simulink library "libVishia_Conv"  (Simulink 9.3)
settings: Solver=ode45  StartTime=0.0  StopTime=10.0  RelTol=1e-3  EnableMultiTasking=on
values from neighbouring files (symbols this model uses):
  Tstep = 0.000050    (= 5e-05)    [TestOrthOsc_init.m]    (also in Test_PIDctrl_init.m = 0.0001)
undefined symbols (not defined in the file or in its folder): b0bit, b1bit, b2bit, b3bit, b4bit, b5bit, b6bit, b7bit, bit, Bitnr, hi, lo, maxFader, val, x0, xnom, y0, ynom
libraries: simulink x2

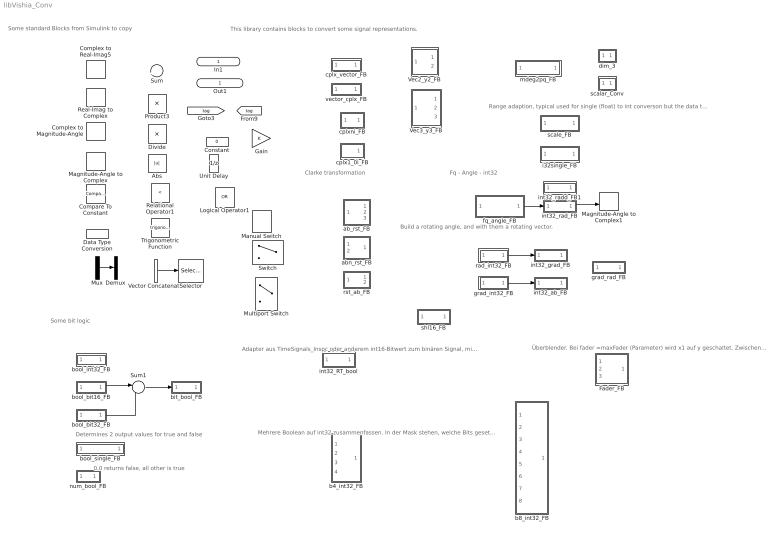
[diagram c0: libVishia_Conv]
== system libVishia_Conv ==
  note: Range adaption, typical used for single (float) to int converson but the data types on input and output depends on connected ones (forward and back propageted). Insert it is a data type conversion element.
  note: Some standard Blocks from Simulink to copy
  note: Mehrere Boolean auf int32 zusammenfassen. In der Mask stehen, welche Bits gesetzt werden. Default ist 0..3 bzw. 0..7, lässt sich ändern.
  note: Überblender. Bei fader =maxFader (Parameter) wird x1 auf y geschaltet. Zwischen diesen Werten überblenden.
  note: Adapter aus TimeSignals_Inspc oder anderem int16-Bitwert zum binären Signal, mit Angabe Bit-Nummer als Parameter. Einschließlich Rate-Transition, Ausgang kann in TstepHw direkt verwendet werden.
  note: This library contains blocks to convert some signal representations.
  note: Determines 2 output values for true and false
  note: 0.0 returns false, all other is true
  note: Clarke transformation
  note: Build a rotating angle, and with them a rotating vector.
  note: Fq - Angle - int32
  note: Some bit logic
  In1 : Inport  OutDataTypeStr=single  PortDimensions=1
  Abs : Abs
  Compare To Constant : simulink/Logic and Bit Operations/Compare To Constant  relop=<=  const=3.0  OutDataTypeStr=boolean
  Complex to Magnitude-Angle : ComplexToMagnitudeAngle
  Complex to Real-Imag5 : ComplexToRealImag
  Constant : Constant  Value=0  OutDataTypeStr=single
  Data Type Conversion : DataTypeConversion  OutDataTypeStr=int32
  Demux : Demux  Outputs=2
  Divide : Product  Inputs=*/
  Fader_FB : Subsystem
  Gain : Gain
  Logical Operator1 : Logic  Operator=OR  IconShape=distinctive  AllPortsSameDT=off  OutDataTypeStr=boolean
  Magnitude-Angle to Complex : MagnitudeAngleToComplex
  Magnitude-Angle to Complex1 : MagnitudeAngleToComplex
  Manual Switch : ManualSwitch
  Multiport Switch : MultiPortSwitch
  Mux : Mux  Inputs=2
  Product3 : Product
  Real-Imag to Complex : RealImagToComplex
  Relational Operator1 : RelationalOperator  Operator=<  OutDataTypeStr=boolean
  Selector : Selector  InputPortWidth=3  IndexOptions=Index vector (dialog)  Indices=[1 3]  OutputSizes=1
  Sum : Sum  Inputs=|++
  Sum1 : Sum  Inputs=|++
  Switch : Switch  Criteria=u2 > Threshold
  Trigonometric Function : Trigonometry
  Unit Delay : UnitDelay  SampleTime=-1  HasFrameUpgradeWarning=on
  Vec2_y2_FB : Subsystem
  Vec3_y3_FB : Subsystem
  Vector Concatenate : Concatenate
  ab_rst_FB : Subsystem
  abn_rst_FB : Subsystem
  b4_int32_FB : Subsystem
  b8_int32_FB : Subsystem
  bit_bool_FB : Subsystem
  bool_bit16_FB : Subsystem
  bool_bit32_FB : Subsystem
  bool_int32_FB : Subsystem
  bool_single_FB : Subsystem
  cplx1_0i_FB : Subsystem
  cplx_vector_FB : Subsystem
  cplxni_FB : Subsystem
  dim_3 : Subsystem
  fq_angle_FB : Subsystem
  grad_int32_FB : Subsystem  TreatAsAtomicUnit=on
  grad_rad_FB : Subsystem
  i32single_FB : Subsystem
  int32_RT_bool : Subsystem
  int32_ab_FB : Subsystem
  int32_grad_FB : Subsystem
  int32_rad_FB : Subsystem
  int32_radd_FB1 : Subsystem
  mdeg2pq_FB : Subsystem
  num_bool_FB : Subsystem
  rad_int32_FB : Subsystem  TreatAsAtomicUnit=on
  rst_ab_FB : Subsystem
  scalar_Conv : Subsystem
  scale_FB : Subsystem
  shl16_FB : Subsystem  TreatAsAtomicUnit=on
  vector_cplx_FB : Subsystem
  Out1 : Outport  OutDataTypeStr=single  PortDimensions=1
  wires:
  int32_rad_FB/1(Out1) -> Magnitude-Angle to Complex1/2
  fq_angle_FB/1(Gint32) -> int32_rad_FB/1(In1)
  rad_int32_FB/1(mwi) -> int32_grad_FB/1(In1)
  grad_int32_FB/1(mwi) -> int32_ab_FB/1(In1)
  Mux/1 -> Demux/1
  Vector Concatenate/1 -> Selector/1
  bool_bit16_FB/1(y) -> Sum1/1
  Sum1/1 -> bit_bool_FB/1(b)
  bool_bit32_FB/1(y) -> Sum1/2

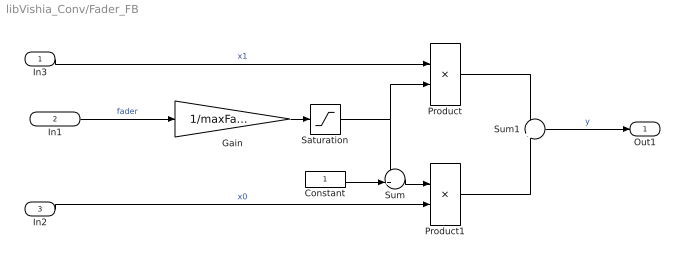
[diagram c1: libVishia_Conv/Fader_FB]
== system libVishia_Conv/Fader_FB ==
  In3 : Inport  OutDataTypeStr=single
  In1 : Inport  Port=2  OutDataTypeStr=single
  In2 : Inport  Port=3  OutDataTypeStr=single
  Constant : Constant  OutDataTypeStr=single
  Gain : Gain  Gain=1/maxFader
  Product : Product
  Product1 : Product
  Saturation : Saturate  UpperLimit=1  LowerLimit=0  ZeroCross=off
  Sum : Sum  Inputs=-+|
  Sum1 : Sum  Inputs=+|+
  Out1 : Outport  OutDataTypeStr=single
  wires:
  In1/1 -> Gain/1  "fader"
  Gain/1 -> Saturation/1
  Saturation/1 -> Product/2, Sum/1
  Constant/1 -> Sum/2
  Sum/1 -> Product1/1
  In2/1 -> Product1/2  "x0"
  In3/1 -> Product/1  "x1"
  Product/1 -> Sum1/1
  Product1/1 -> Sum1/2
  Sum1/1 -> Out1/1  "y"

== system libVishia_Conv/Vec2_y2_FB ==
  In1 : Inport  PortDimensions=2
  Selector : Selector  IndexMode=Zero-based  InputPortWidth=2  IndexOptions=Index vector (dialog)  Indices=[0]  OutputSizes=1
  Selector1 : Selector  IndexMode=Zero-based  InputPortWidth=2  IndexOptions=Index vector (dialog)  Indices=[1]  OutputSizes=1
  Out1 : Outport
  Out2 : Outport  Port=2
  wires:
  Selector1/1 -> Out2/1  "y1"
  In1/1 -> Selector1/1, Selector/1
  Selector/1 -> Out1/1  "y0"

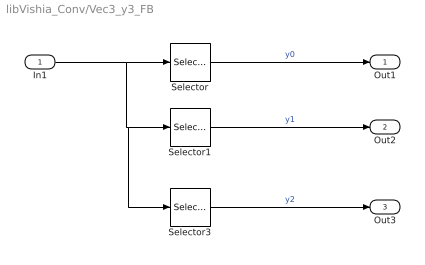
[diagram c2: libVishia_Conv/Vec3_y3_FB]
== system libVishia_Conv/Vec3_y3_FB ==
  In1 : Inport  PortDimensions=3
  Selector : Selector  IndexMode=Zero-based  InputPortWidth=3  IndexOptions=Index vector (dialog)  Indices=[0]  OutputSizes=1
  Selector1 : Selector  IndexMode=Zero-based  InputPortWidth=3  IndexOptions=Index vector (dialog)  Indices=[1]  OutputSizes=1
  Selector3 : Selector  IndexMode=Zero-based  InputPortWidth=3  IndexOptions=Index vector (dialog)  Indices=[2]  OutputSizes=1
  Out1 : Outport
  Out2 : Outport  Port=2
  Out3 : Outport  Port=3
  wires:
  Selector/1 -> Out1/1  "y0"
  In1/1 -> Selector/1, Selector3/1, Selector1/1
  Selector1/1 -> Out2/1  "y1"
  Selector3/1 -> Out3/1  "y2"

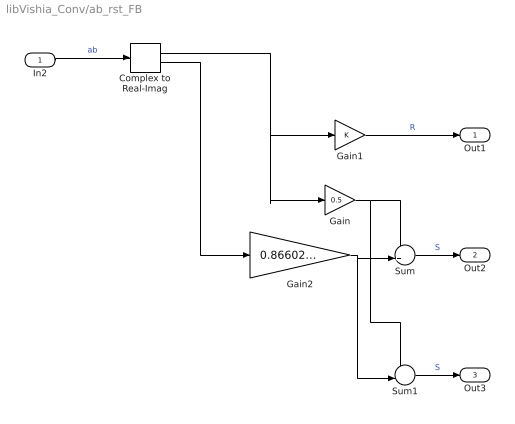
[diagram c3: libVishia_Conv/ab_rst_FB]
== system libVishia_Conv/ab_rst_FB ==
  In2 : Inport  OutDataTypeStr=single
  Complex to Real-Imag : ComplexToRealImag
  Gain : Gain  Gain=0.5
  Gain1 : Gain
  Gain2 : Gain  Gain=0.86602540
  Sum : Sum  Inputs=-+|
  Sum1 : Sum  Inputs=--|
  Out1 : Outport
  Out2 : Outport  Port=2
  Out3 : Outport  Port=3
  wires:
  Sum1/1 -> Out3/1  "S"
  Gain/1 -> Sum/1, Sum1/1
  Complex to Real-Imag/2 -> Gain2/1
  Gain2/1 -> Sum/2, Sum1/2
  In2/1 -> Complex to Real-Imag/1  "ab"
  Gain1/1 -> Out1/1  "R"
  Complex to Real-Imag/1 -> Gain1/1, Gain/1
  Sum/1 -> Out2/1  "S"

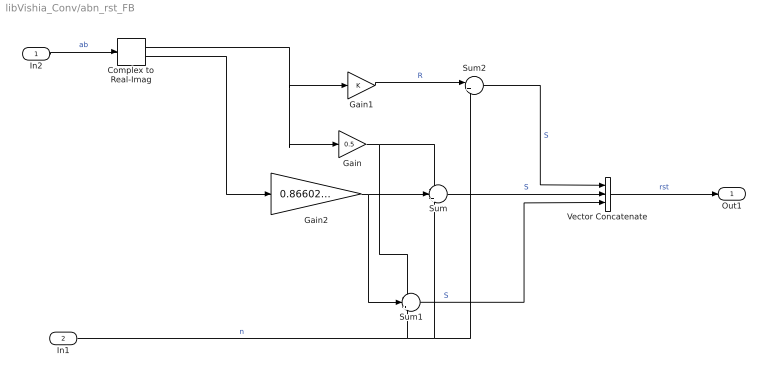
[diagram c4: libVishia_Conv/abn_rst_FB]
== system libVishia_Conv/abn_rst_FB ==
  In2 : Inport  PortDimensions=1
  In1 : Inport  Port=2
  Complex to Real-Imag : ComplexToRealImag
  Gain : Gain  Gain=0.5
  Gain1 : Gain
  Gain2 : Gain  Gain=0.86602540
  Sum : Sum  Inputs=-++
  Sum1 : Sum  Inputs=--+
  Sum2 : Sum  Inputs=|++
  Vector Concatenate : Concatenate  NumInputs=3
  Out1 : Outport  PortDimensions=3
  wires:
  Sum2/1 -> Vector Concatenate/1  "S"
  In1/1 -> Sum1/3, Sum/3, Sum2/2  "n"
  Vector Concatenate/1 -> Out1/1  "rst"
  Sum1/1 -> Vector Concatenate/3  "S"
  Gain/1 -> Sum/1, Sum1/1
  Complex to Real-Imag/2 -> Gain2/1
  Gain2/1 -> Sum/2, Sum1/2
  In2/1 -> Complex to Real-Imag/1  "ab"
  Gain1/1 -> Sum2/1  "R"
  Complex to Real-Imag/1 -> Gain1/1, Gain/1
  Sum/1 -> Vector Concatenate/2  "S"

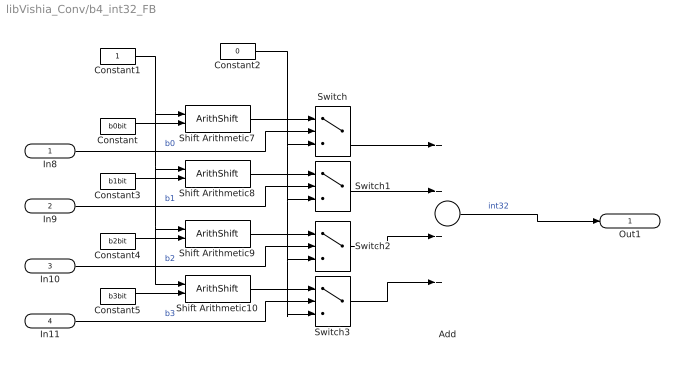
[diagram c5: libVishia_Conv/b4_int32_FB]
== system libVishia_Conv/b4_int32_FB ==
  In8 : Inport  OutDataTypeStr=boolean
  In9 : Inport  Port=2  OutDataTypeStr=boolean
  In10 : Inport  Port=3  OutDataTypeStr=boolean
  In11 : Inport  Port=4  OutDataTypeStr=boolean
  Add : Sum  Inputs=++++
  Constant : Constant  Value=b0bit  OutDataTypeStr=uint32
  Constant1 : Constant  OutDataTypeStr=uint32
  Constant2 : Constant  Value=0  OutDataTypeStr=uint32
  Constant3 : Constant  Value=b1bit  OutDataTypeStr=uint32
  Constant4 : Constant  Value=b2bit  OutDataTypeStr=uint32
  Constant5 : Constant  Value=b3bit  OutDataTypeStr=uint32
  Shift Arithmetic{7..10} (4 alike) : ArithShift  BitShiftNumberSource=Input port  BitShiftNumber=6  BitShiftDirection=Left
  Switch{,1..3} (4 alike) : Switch  Criteria=u2 ~= 0  OutDataTypeStr=uint32
  Out1 : Outport  OutDataTypeStr=uint32  PortDimensions=1
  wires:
  In8/1 -> Switch/2  "b0"
  Add/1 -> Out1/1  "int32"
  Constant/1 -> Shift Arithmetic7/2
  Shift Arithmetic7/1 -> Switch/1
  Constant1/1 -> Shift Arithmetic10/1, Shift Arithmetic9/1, Shift Arithmetic8/1, Shift Arithmetic7/1
  Constant2/1 -> Switch1/3, Switch3/3, Switch2/3, Switch/3
  In9/1 -> Switch1/2  "b1"
  Constant3/1 -> Shift Arithmetic8/2
  Shift Arithmetic8/1 -> Switch1/1
  In10/1 -> Switch2/2  "b2"
  Constant4/1 -> Shift Arithmetic9/2
  Shift Arithmetic9/1 -> Switch2/1
  In11/1 -> Switch3/2  "b3"
  Constant5/1 -> Shift Arithmetic10/2
  Shift Arithmetic10/1 -> Switch3/1
  Switch/1 -> Add/1
  Switch1/1 -> Add/2
  Switch2/1 -> Add/3
  Switch3/1 -> Add/4

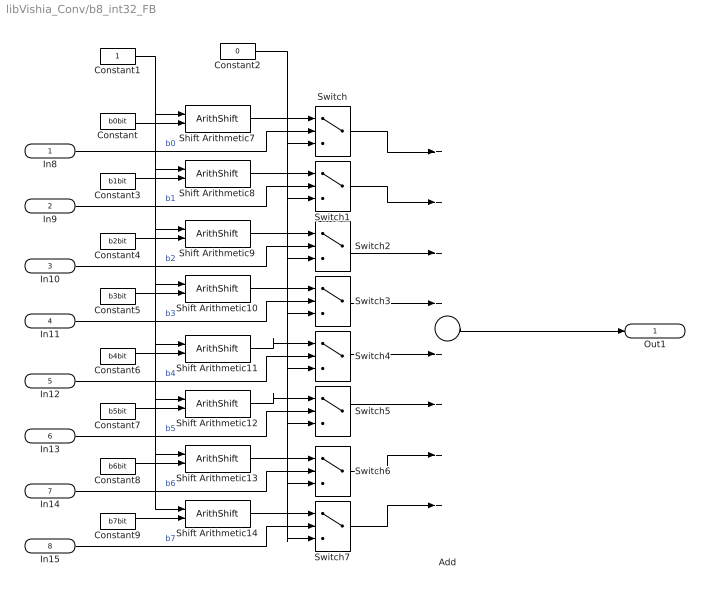
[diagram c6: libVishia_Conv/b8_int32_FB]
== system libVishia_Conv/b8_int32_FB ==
  In8 : Inport  OutDataTypeStr=boolean
  In9 : Inport  Port=2  OutDataTypeStr=boolean
  In10 : Inport  Port=3  OutDataTypeStr=boolean
  In11 : Inport  Port=4  OutDataTypeStr=boolean
  In12 : Inport  Port=5  OutDataTypeStr=boolean
  In13 : Inport  Port=6  OutDataTypeStr=boolean
  In14 : Inport  Port=7  OutDataTypeStr=boolean
  In15 : Inport  Port=8  OutDataTypeStr=boolean
  Add : Sum  Inputs=++++++++
  Constant : Constant  Value=b0bit  OutDataTypeStr=uint32
  Constant1 : Constant  OutDataTypeStr=uint32
  Constant2 : Constant  Value=0  OutDataTypeStr=uint32
  Constant3 : Constant  Value=b1bit  OutDataTypeStr=uint32
  Constant4 : Constant  Value=b2bit  OutDataTypeStr=uint32
  Constant5 : Constant  Value=b3bit  OutDataTypeStr=uint32
  Constant6 : Constant  Value=b4bit  OutDataTypeStr=uint32
  Constant7 : Constant  Value=b5bit  OutDataTypeStr=uint32
  Constant8 : Constant  Value=b6bit  OutDataTypeStr=uint32
  Constant9 : Constant  Value=b7bit  OutDataTypeStr=uint32
  Shift Arithmetic{7..14} (8 alike) : ArithShift  BitShiftNumberSource=Input port  BitShiftNumber=6  BitShiftDirection=Left
  Switch{,1..7} (8 alike) : Switch  Criteria=u2 ~= 0  OutDataTypeStr=uint32
  Out1 : Outport  OutDataTypeStr=uint32  PortDimensions=1
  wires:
  In8/1 -> Switch/2  "b0"
  Constant/1 -> Shift Arithmetic7/2
  Shift Arithmetic7/1 -> Switch/1
  Constant1/1 -> Shift Arithmetic14/1, Shift Arithmetic13/1, Shift Arithmetic12/1, Shift Arithmetic11/1, Shift Arithmetic10/1, Shift Arithmetic9/1, Shift Arithmetic8/1, Shift Arithmetic7/1
  Constant2/1 -> Switch/3, Switch1/3, Switch2/3, Switch3/3, Switch6/3, Switch7/3, Switch5/3, Switch4/3
  In9/1 -> Switch1/2  "b1"
  Constant3/1 -> Shift Arithmetic8/2
  Shift Arithmetic8/1 -> Switch1/1
  In10/1 -> Switch2/2  "b2"
  Constant4/1 -> Shift Arithmetic9/2
  Shift Arithmetic9/1 -> Switch2/1
  In11/1 -> Switch3/2  "b3"
  Constant5/1 -> Shift Arithmetic10/2
  Shift Arithmetic10/1 -> Switch3/1
  In12/1 -> Switch4/2  "b4"
  Constant6/1 -> Shift Arithmetic11/2
  Shift Arithmetic11/1 -> Switch4/1
  In13/1 -> Switch5/2  "b5"
  Constant7/1 -> Shift Arithmetic12/2
  Shift Arithmetic12/1 -> Switch5/1
  In14/1 -> Switch6/2  "b6"
  Constant8/1 -> Shift Arithmetic13/2
  Shift Arithmetic13/1 -> Switch6/1
  In15/1 -> Switch7/2  "b7"
  Constant9/1 -> Shift Arithmetic14/2
  Shift Arithmetic14/1 -> Switch7/1
  Switch/1 -> Add/1
  Switch1/1 -> Add/2
  Switch2/1 -> Add/3
  Switch3/1 -> Add/4
  Switch7/1 -> Add/8
  Switch6/1 -> Add/7
  Switch5/1 -> Add/6
  Switch4/1 -> Add/5
  Add/1 -> Out1/1

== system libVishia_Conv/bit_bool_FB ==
  b : Inport
  Constant : Constant  Value=bitshift(1, bit)  OutDataTypeStr=Inherit: Inherit via back propagation
  Data Type Duplicate : DataTypeDuplicate
  Logical Operator : Logic  AllPortsSameDT=off  OutDataTypeStr=boolean
  y : Outport  OutDataTypeStr=boolean
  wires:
  Logical Operator/1 -> y/1
  b/1 -> Data Type Duplicate/1, Logical Operator/1  "b"
  Constant/1 -> Data Type Duplicate/2, Logical Operator/2

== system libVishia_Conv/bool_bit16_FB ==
  b : Inport  OutDataTypeStr=boolean
  Constant : Constant  Value=bitshift(1, bit)  OutDataTypeStr=uint16
  Constant1 : Constant  Value=0  OutDataTypeStr=uint16
  Switch : Switch  Criteria=u2 ~= 0  OutDataTypeStr=Inherit: Inherit via back propagation
  y : Outport
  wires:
  Constant/1 -> Switch/1
  Constant1/1 -> Switch/3
  b/1 -> Switch/2  "b"
  Switch/1 -> y/1

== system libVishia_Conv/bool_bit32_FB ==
  b : Inport  OutDataTypeStr=boolean
  Constant : Constant  Value=bitshift(1, bit)  OutDataTypeStr=uint32
  Constant1 : Constant  Value=0  OutDataTypeStr=uint32
  Switch : Switch  Criteria=u2 ~= 0  OutDataTypeStr=Inherit: Inherit via back propagation
  y : Outport
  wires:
  Switch/1 -> y/1
  b/1 -> Switch/2  "b"
  Constant1/1 -> Switch/3
  Constant/1 -> Switch/1

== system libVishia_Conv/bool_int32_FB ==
  b : Inport
  Constant : Constant  Value=val  OutDataTypeStr=int32
  Constant1 : Constant  Value=0  OutDataTypeStr=int32
  Switch : Switch  Criteria=u2 ~= 0  OutDataTypeStr=int32
  y : Outport  OutDataTypeStr=int32
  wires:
  Switch/1 -> y/1
  b/1 -> Switch/2  "b"
  Constant1/1 -> Switch/3
  Constant/1 -> Switch/1

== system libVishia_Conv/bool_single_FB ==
  b : Inport
  Constant : Constant  Value=hi  OutDataTypeStr=Inherit: Inherit via back propagation
  Constant1 : Constant  Value=lo  OutDataTypeStr=Inherit: Inherit via back propagation
  Switch : Switch  Criteria=u2 ~= 0
  y : Outport
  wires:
  Constant/1 -> Switch/1
  Constant1/1 -> Switch/3
  b/1 -> Switch/2  "b"
  Switch/1 -> y/1

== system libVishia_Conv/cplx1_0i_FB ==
  Constant : Constant  OutDataTypeStr=Inherit: Inherit via back propagation
  Constant1 : Constant  Value=0  OutDataTypeStr=Inherit: Inherit via back propagation
  Real-Imag to Complex : RealImagToComplex
  Out1 : Outport
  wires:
  Real-Imag to Complex/1 -> Out1/1  "1+0i"
  Constant/1 -> Real-Imag to Complex/1
  Constant1/1 -> Real-Imag to Complex/2

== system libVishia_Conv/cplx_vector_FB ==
  In1 : Inport  PortDimensions=1
  Complex to Real-Imag : ComplexToRealImag
  Vector Concatenate : Concatenate
  Out1 : Outport  PortDimensions=2
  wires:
  Complex to Real-Imag/1 -> Vector Concatenate/1
  Complex to Real-Imag/2 -> Vector Concatenate/2
  In1/1 -> Complex to Real-Imag/1
  Vector Concatenate/1 -> Out1/1  "dqV"

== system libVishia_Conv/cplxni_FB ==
  In1 : Inport  OutDataTypeStr=single
  Complex to Real-Imag : ComplexToRealImag
  Gain : Gain  Gain=-1
  Real-Imag to Complex : RealImagToComplex
  Out1 : Outport  OutDataTypeStr=single
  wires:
  In1/1 -> Complex to Real-Imag/1  "ri"
  Complex to Real-Imag/1 -> Real-Imag to Complex/1
  Real-Imag to Complex/1 -> Out1/1  "rni"
  Complex to Real-Imag/2 -> Gain/1
  Gain/1 -> Real-Imag to Complex/2

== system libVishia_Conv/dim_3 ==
  In1 : Inport  PortDimensions=3
  Out1 : Outport  PortDimensions=3
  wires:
  In1/1 -> Out1/1  "3"

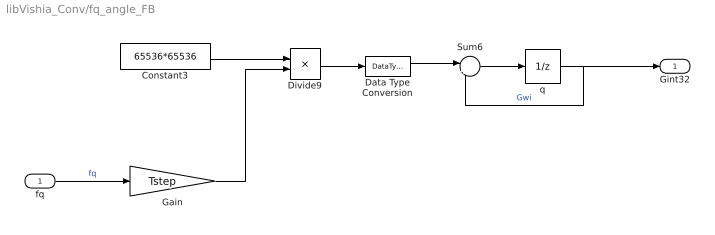
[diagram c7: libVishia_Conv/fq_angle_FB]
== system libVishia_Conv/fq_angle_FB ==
  fq : Inport
  Constant3 : Constant  Value=65536*65536  OutDataTypeStr=single
  Data Type Conversion : DataTypeConversion  OutDataTypeStr=int32
  Divide9 : Product  Inputs=**
  Gain : Gain  Gain=Tstep
  Sum6 : Sum  Inputs=|++
  q : UnitDelay  SampleTime=Tstep  HasFrameUpgradeWarning=on
  Gint32 : Outport
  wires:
  Data Type Conversion/1 -> Sum6/1
  Sum6/1 -> q/1
  q/1 -> Gint32/1, Sum6/2  "Gwi"
  Constant3/1 -> Divide9/1
  Gain/1 -> Divide9/2
  fq/1 -> Gain/1  "fq"
  Divide9/1 -> Data Type Conversion/1

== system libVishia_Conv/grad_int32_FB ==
  pq : Inport
  Data Type Conversion : DataTypeConversion  OutDataTypeStr=int32  RndMeth=Simplest
  Gain2 : Gain  Gain=65536*32768 / 180
  mwi : Outport  OutDataTypeStr=int32
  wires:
  Data Type Conversion/1 -> mwi/1  "int"
  Gain2/1 -> Data Type Conversion/1
  pq/1 -> Gain2/1  "grad"

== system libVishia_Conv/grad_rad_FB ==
  In1 : Inport
  Gain : Gain  Gain=pi/180
  Out1 : Outport
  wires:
  In1/1 -> Gain/1  "grad"
  Gain/1 -> Out1/1  "rad"

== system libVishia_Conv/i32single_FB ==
  In1 : Inport  OutDataTypeStr=int32
  Data Type Conversion1 : DataTypeConversion  OutDataTypeStr=single
  Gain : Gain  Gain=ynom/(32768*65536)
  Out1 : Outport
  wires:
  Data Type Conversion1/1 -> Gain/1  "y"
  Gain/1 -> Out1/1  "y"
  In1/1 -> Data Type Conversion1/1  "x"

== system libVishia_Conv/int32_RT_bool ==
  In1 : Inport  OutDataTypeStr=int16
  Bitwise Operator : simulink/Logic and Bit Operations/Bitwise Operator  logicop=AND  UseBitMask=on  BitMask=bitshift(1,Bitnr)  BitMaskRealWorld=Stored Integer
  Data Type Conversion : DataTypeConversion  OutDataTypeStr=boolean
  Rate Transition7 : RateTransition  OutPortSampleTime=TstepHw
  Out1 : Outport  OutDataTypeStr=boolean
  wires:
  Data Type Conversion/1 -> Rate Transition7/1
  Bitwise Operator/1 -> Data Type Conversion/1
  In1/1 -> Bitwise Operator/1  "x16_RT"
  Rate Transition7/1 -> Out1/1  "bin"

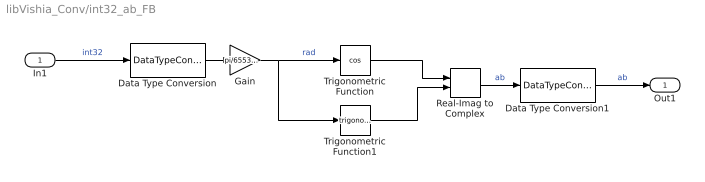
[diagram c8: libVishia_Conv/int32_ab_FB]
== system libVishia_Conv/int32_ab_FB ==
  In1 : Inport
  Data Type Conversion : DataTypeConversion  OutDataTypeStr=single
  Data Type Conversion1 : DataTypeConversion  OutDataTypeStr=single
  Gain : Gain  Gain=pi/65536/32768
  Real-Imag to Complex : RealImagToComplex
  Trigonometric Function : Trigonometry  Operator=cos
  Trigonometric Function1 : Trigonometry
  Out1 : Outport  OutDataTypeStr=single
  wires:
  Data Type Conversion1/1 -> Out1/1  "ab"
  Real-Imag to Complex/1 -> Data Type Conversion1/1  "ab"
  Trigonometric Function1/1 -> Real-Imag to Complex/2
  Trigonometric Function/1 -> Real-Imag to Complex/1
  In1/1 -> Data Type Conversion/1  "int32"
  Gain/1 -> Trigonometric Function/1, Trigonometric Function1/1  "rad"
  Data Type Conversion/1 -> Gain/1

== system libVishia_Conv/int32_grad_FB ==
  In1 : Inport
  Data Type Conversion : DataTypeConversion  OutDataTypeStr=single
  Gain : Gain  Gain=180/65536/32768
  Out1 : Outport
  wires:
  Data Type Conversion/1 -> Gain/1
  Gain/1 -> Out1/1  "grad"
  In1/1 -> Data Type Conversion/1  "int32"

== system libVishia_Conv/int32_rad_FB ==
  In1 : Inport
  Data Type Conversion : DataTypeConversion  OutDataTypeStr=single
  Gain : Gain  Gain=pi/65536/32768
  Out1 : Outport
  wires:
  In1/1 -> Data Type Conversion/1  "int32"
  Gain/1 -> Out1/1  "rad"
  Data Type Conversion/1 -> Gain/1

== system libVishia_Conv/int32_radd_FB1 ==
  In1 : Inport
  Data Type Conversion : DataTypeConversion  OutDataTypeStr=double
  Gain : Gain  Gain=pi/65536/32768
  Out1 : Outport
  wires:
  In1/1 -> Data Type Conversion/1  "int32"
  Gain/1 -> Out1/1  "rad"
  Data Type Conversion/1 -> Gain/1

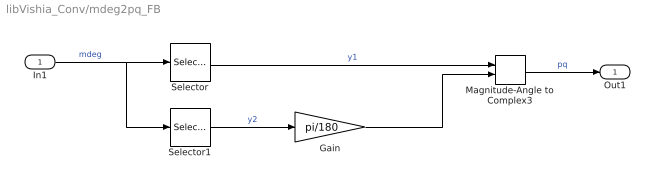
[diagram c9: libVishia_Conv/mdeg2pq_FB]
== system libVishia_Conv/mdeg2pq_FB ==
  In1 : Inport  PortDimensions=2
  Gain : Gain  Gain=pi/180
  Magnitude-Angle to Complex3 : MagnitudeAngleToComplex
  Selector : Selector  IndexMode=Zero-based  InputPortWidth=2  IndexOptions=Index vector (dialog)  Indices=[0]  OutputSizes=1
  Selector1 : Selector  IndexMode=Zero-based  InputPortWidth=2  IndexOptions=Index vector (dialog)  Indices=[1]  OutputSizes=1
  Out1 : Outport
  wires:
  Selector1/1 -> Gain/1  "y2"
  In1/1 -> Selector1/1, Selector/1  "mdeg"
  Magnitude-Angle to Complex3/1 -> Out1/1  "pq"
  Selector/1 -> Magnitude-Angle to Complex3/1  "y1"
  Gain/1 -> Magnitude-Angle to Complex3/2

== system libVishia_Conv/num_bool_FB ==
  x : Inport
  Constant1 : Constant  Value=0  OutDataTypeStr=single
  Relational Operator : RelationalOperator  Operator=>  OutDataTypeStr=boolean
  b : Outport
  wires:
  Relational Operator/1 -> b/1
  Constant1/1 -> Relational Operator/2
  x/1 -> Relational Operator/1

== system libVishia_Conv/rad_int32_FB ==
  pq : Inport
  Data Type Conversion : DataTypeConversion  OutDataTypeStr=int32  RndMeth=Simplest
  Gain2 : Gain  Gain=65536*32768 / pi
  mwi : Outport
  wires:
  pq/1 -> Gain2/1  "rad"
  Gain2/1 -> Data Type Conversion/1
  Data Type Conversion/1 -> mwi/1  "in32"

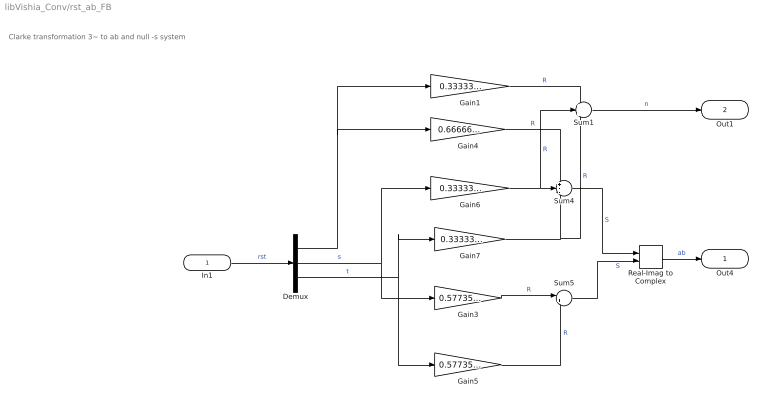
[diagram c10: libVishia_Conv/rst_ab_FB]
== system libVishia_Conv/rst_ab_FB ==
  note: Clarke transformation 3~ to ab and null -s system
  In1 : Inport  PortDimensions=3
  Demux : Demux  Outputs=3
  Gain1 : Gain  Gain=0.3333333
  Gain3 : Gain  Gain=0.5773503
  Gain4 : Gain  Gain=0.6666667
  Gain5 : Gain  Gain=0.5773503
  Gain6 : Gain  Gain=0.3333333
  Gain7 : Gain  Gain=0.3333333
  Real-Imag to Complex : RealImagToComplex
  Sum1 : Sum  Inputs=+++
  Sum4 : Sum  Inputs=+--
  Sum5 : Sum  Inputs=|+-
  Out4 : Outport
  Out1 : Outport  Port=2
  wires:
  Sum1/1 -> Out1/1  "n"
  Gain1/1 -> Sum1/1  "R"
  Demux/1 -> Gain4/1, Gain1/1
  Real-Imag to Complex/1 -> Out4/1  "ab"
  Gain5/1 -> Sum5/2  "R"
  Gain3/1 -> Sum5/1  "R"
  Gain7/1 -> Sum4/3, Sum1/3  "R"
  Gain6/1 -> Sum1/2, Sum4/2  "R"
  Sum5/1 -> Real-Imag to Complex/2  "S"
  Sum4/1 -> Real-Imag to Complex/1  "S"
  Gain4/1 -> Sum4/1  "R"
  Demux/3 -> Gain7/1, Gain5/1  "t"
  Demux/2 -> Gain3/1, Gain6/1  "s"
  In1/1 -> Demux/1  "rst"

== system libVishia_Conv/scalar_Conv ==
  In1 : Inport
  Out1 : Outport  PortDimensions=1
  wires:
  In1/1 -> Out1/1  "1"

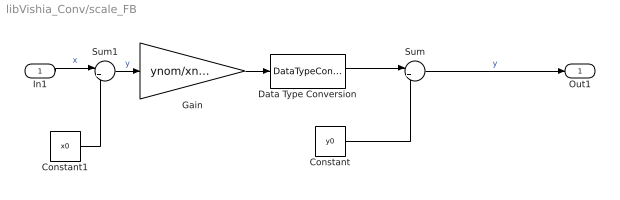
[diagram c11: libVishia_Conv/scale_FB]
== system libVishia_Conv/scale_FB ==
  In1 : Inport
  Constant : Constant  Value=y0  OutDataTypeStr=Inherit: Inherit via back propagation
  Constant1 : Constant  Value=x0  OutDataTypeStr=Inherit: Inherit via back propagation
  Data Type Conversion : DataTypeConversion
  Gain : Gain  Gain=ynom/xnom
  Sum : Sum  Inputs=|++
  Sum1 : Sum  Inputs=|+-
  Out1 : Outport
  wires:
  In1/1 -> Sum1/1  "x"
  Gain/1 -> Data Type Conversion/1
  Sum/1 -> Out1/1  "y"
  Constant/1 -> Sum/2
  Data Type Conversion/1 -> Sum/1
  Sum1/1 -> Gain/1  "y"
  Constant1/1 -> Sum1/2

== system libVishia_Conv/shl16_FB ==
  pq : Inport
  Data Type Conversion1 : DataTypeConversion  OutDataTypeStr=int32  RndMeth=Simplest
  Gain2 : Gain  Gain=65536  OutDataTypeStr=int32
  mwi : Outport  OutDataTypeStr=int32
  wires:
  pq/1 -> Data Type Conversion1/1  "i16"
  Gain2/1 -> mwi/1  "i32"
  Data Type Conversion1/1 -> Gain2/1

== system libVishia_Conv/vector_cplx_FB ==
  In1 : Inport  PortDimensions=2
  Real-Imag to Complex : RealImagToComplex
  Selector : Selector  IndexMode=Zero-based  InputPortWidth=2  IndexOptions=Index vector (dialog)  Indices=[0]  OutputSizes=1
  Selector1 : Selector  IndexMode=Zero-based  InputPortWidth=2  IndexOptions=Index vector (dialog)  Indices=[1]  OutputSizes=1
  Out1 : Outport
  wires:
  Selector1/1 -> Real-Imag to Complex/2
  Real-Imag to Complex/1 -> Out1/1  "ri"
  Selector/1 -> Real-Imag to Complex/1
  In1/1 -> Selector1/1, Selector/1
